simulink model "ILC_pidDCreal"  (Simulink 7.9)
settings: Solver=ode1  SolverMode=SingleTasking  StartTime=time_ILC(1)  StopTime=time_ILC(end)  FixedStep=tsamp_ILC  RelTol=1e-3  AbsTol=1e-6
PreLoadFcn:
  | ILC_setup
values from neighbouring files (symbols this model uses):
  Ts = 0.1    [pidDCinit.m]    (also in stupidDCinit.m; da_bode_evolution.m = 1)
  tsamp_ILC = 0.010    (= 0.01)    [ILC_setup.m]
undefined symbols (not defined in the file or in its folder): DiscIntNeverNeededParam

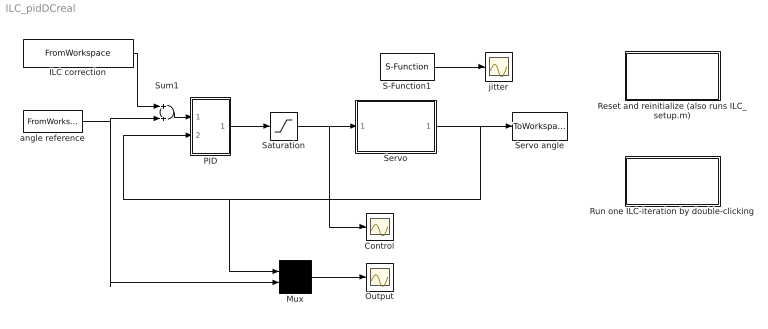
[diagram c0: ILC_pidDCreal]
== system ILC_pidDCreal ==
  Control : Scope
  ILC correction : FromWorkspace  VariableName=[ time_ILC correction_ILC(:,idx_ILC)]  SampleTime=tsamp_ILC
  Mux : Mux  Inputs=2
  Output : Scope
  PID : Subsystem  mask{K=1.7, Ti=0.8, Td=0.3}
      mask init:
      | b_reg=1; c_reg=0;
  Reset and reinitialize (also runs ILC_setup.m) : Subsystem
  Run one ILC-iteration by double-clicking : Subsystem
  S-Function1 : S-Function  FunctionName=realtimer  Parameters=tsamp_ILC  EnableBusSupport=off
  Saturation : Saturate  UpperLimit=10  LowerLimit=-10
  Servo : Subsystem
  Servo angle : ToWorkspace  VariableName=ILC_pos  SampleTime=-1  SaveFormat=Structure With Time
  Sum1 : Sum
  angle reference : FromWorkspace  VariableName=[ time_ILC pos_Reference_ILC]  SampleTime=tsamp_ILC
  jitter : Scope
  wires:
  Mux/1 -> Output/1
  angle reference/1 -> Mux/2, Sum1/2
  PID/1(Out1) -> Saturation/1
  Servo/1(p_2) -> Mux/1, PID/2(y), Servo angle/1
  S-Function1/1 -> jitter/1
  Saturation/1 -> Servo/1(u), Control/1
  Sum1/1 -> PID/1(uc)
  ILC correction/1 -> Sum1/1

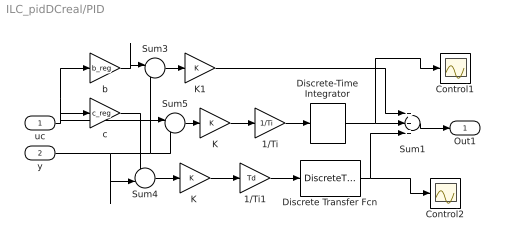
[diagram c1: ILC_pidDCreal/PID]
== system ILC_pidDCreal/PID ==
  uc : Inport
  y : Inport  Port=2
  1/Ti : Gain  Gain=1/Ti
  1/Ti1 : Gain  Gain=Td
  Control1 : Scope
  Control2 : Scope
  Discrete Transfer Fcn : DiscreteTransferFcn  Numerator=[1 -1]*1/(Td/10+Ts)  Denominator=[1 -Td/(Td+10*Ts)]  SampleTime=Ts
  Discrete-Time Integrator : DiscreteIntegrator  SampleTime=Ts  ICPrevOutput=DiscIntNeverNeededParam  ICPrevScaledInput=DiscIntNeverNeededParam
  K : Gain  Gain=K
  "K " : Gain  Gain=K
  K1 : Gain  Gain=K
  Sum1 : Sum  Inputs=+++
  Sum3 : Sum  Inputs=+-
  Sum4 : Sum  Inputs=+-
  Sum5 : Sum  Inputs=+-
  b : Gain  Gain=b_reg
  c : Gain  Gain=c_reg
  Out1 : Outport
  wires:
  K/1 -> 1/Ti/1
  1/Ti/1 -> Discrete-Time Integrator/1
  Sum1/1 -> Out1/1
  Discrete-Time Integrator/1 -> Sum1/2, Control1/1
  Discrete Transfer Fcn/1 -> Sum1/3, Control2/1
  1/Ti1/1 -> Discrete Transfer Fcn/1
  "K "/1 -> 1/Ti1/1
  uc/1 -> c/1, b/1, Sum5/1
  b/1 -> Sum3/1
  y/1 -> Sum4/2, Sum3/2, Sum5/2
  Sum3/1 -> K1/1
  K1/1 -> Sum1/1
  c/1 -> Sum4/1
  Sum4/1 -> "K "/1
  Sum5/1 -> K/1

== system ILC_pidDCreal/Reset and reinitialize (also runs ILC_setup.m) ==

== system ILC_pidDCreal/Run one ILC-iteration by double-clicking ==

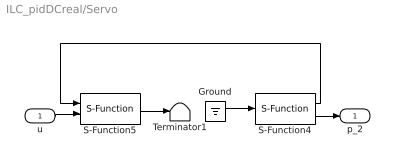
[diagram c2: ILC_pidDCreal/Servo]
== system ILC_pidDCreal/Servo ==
  u : Inport
  Ground : Ground
  S-Function4 : S-Function  FunctionName=analogin  Parameters=tsamp_ILC [0]  EnableBusSupport=off
  S-Function5 : S-Function  FunctionName=analogout  Parameters=tsamp_ILC [0]  EnableBusSupport=off
  Terminator1 : Terminator
  p_2 : Outport
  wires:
  Ground/1 -> S-Function4/1
  S-Function5/1 -> Terminator1/1
  S-Function4/1 -> S-Function5/1
  S-Function4/2 -> p_2/1
  u/1 -> S-Function5/2
